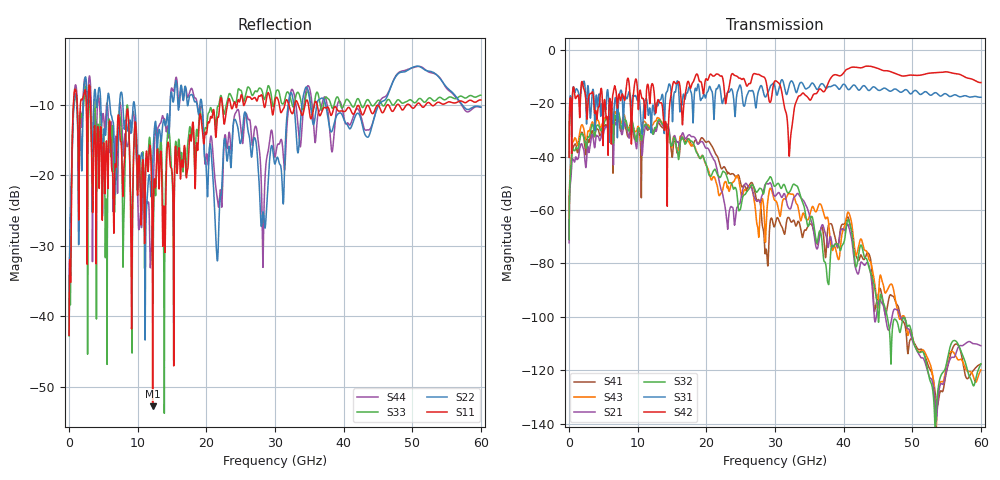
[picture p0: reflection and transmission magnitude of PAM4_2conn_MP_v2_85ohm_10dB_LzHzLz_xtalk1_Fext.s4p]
! Info: Touchstone file created by Circ.  Input file=FAB50GbE_2conn_Midplane_Examax_Topo2_v2_85ohm_10dB_LzHzLz.circ
# Hz S RI R 50
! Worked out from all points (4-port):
!   6000 points, 10 MHz to 60 GHz, reference 50 ohm
!   strongest paths, dB at 10 MHz, 15.01 GHz, 30.01 GHz, 45.01 GHz, 60 GHz:
!     S42: -40.3, -14.5, -11.7, -7.0, -12.3
!     S31: -40.0, -23.2, -14.0, -15.1, -17.8
!     S32: -71.1, -35.9, -51.1, -99.9, -117.6
!     S21: -72.3, -35.4, -54.8, -95.7, -110.9
!     S43: -71.0, -36.2, -56.5, -95.0, -119.9
!     S41: -67.6, -40.2, -65.6, -92.1, -117.7
!   lowest |S11| = -52.8 dB at 12.18 GHz (marker M1), VSWR 1.00, Z = 49.8 - j0.101 ohm
!   |S11| at or under -10 dB: 3.138 GHz to 21.96 GHz (18.82 GHz wide, 150 % of centre); 36.15 GHz to 46.38 GHz (10.23 GHz wide, 24.8 % of centre); 46.49 GHz to 47.78 GHz (1.288 GHz wide, 2.73 % of centre)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
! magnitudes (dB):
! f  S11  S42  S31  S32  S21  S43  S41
! 10 MHz  -42.7  -40.3  -40.0  -71.1  -72.3  -71.0  -67.6
! 890 MHz  -7.8  -18.0  -15.9  -37.6  -41.1  -33.1  -35.3
! 12.18 GHz  -52.8  -12.9  -21.0  -31.5  -30.6  -28.2  -30.2
! 26.66 GHz  -9.2  -10.4  -15.2  -50.6  -52.2  -51.9  -49.8
! 28.79 GHz  -9.0  -13.0  -17.0  -49.6  -50.2  -61.5  -75.9
! 37.5 GHz  -10.5  -14.1  -14.5  -82.4  -70.2  -63.0  -73.9
! 60 GHz  -9.3  -12.3  -17.8  -117.6  -110.9  -119.9  -117.7
